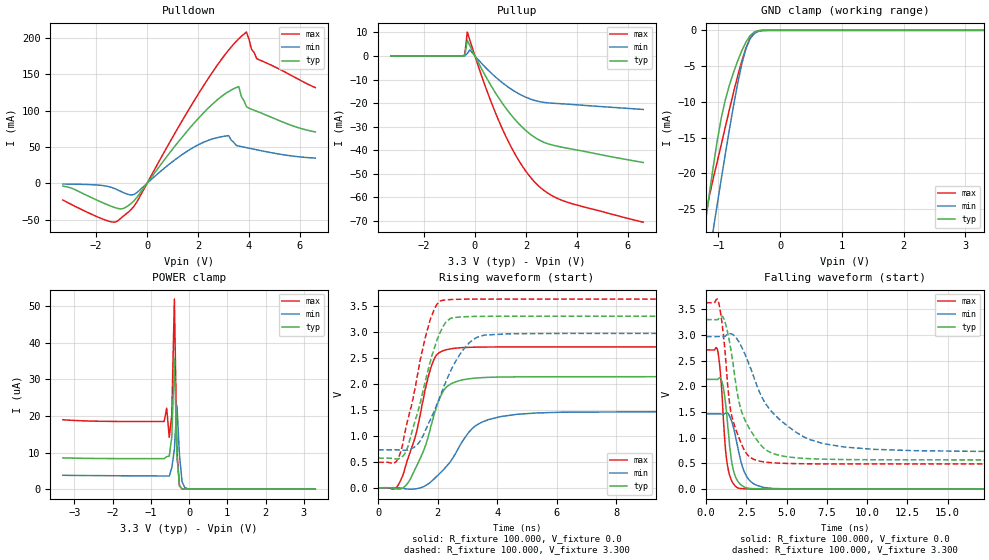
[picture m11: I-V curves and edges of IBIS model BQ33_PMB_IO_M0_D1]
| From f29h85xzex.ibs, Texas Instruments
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|   Model BQ33_PMB_IO_M0_D1
[Model]   BQ33_PMB_IO_M0_D1
Model_type   I/O
Polarity   Non-Inverting
Enable   Active-Low
Vinl =   0.990V
Vinh =   2.310V
Vmeas =  1.650V
Cref =   100.000pF
Vref =   0.0V
|   typ   min   max
C_comp   1.646pF   1.624pF   1.799pF
[Model Spec]
Vinh   2.310V   2.079V   2.541V
Vinl   0.990V   0.891V   1.089V
[Temperature Range]   30   155   -40
[Voltage Range]   3.300V   2.970V   3.630V
[Pullup Reference]   3.300V   2.970V   3.630V
[Pulldown Reference]   0.0V   0.0V   0.0V
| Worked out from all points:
|   slope of the pulldown table from 0 to 0.495 V, typ, clamps not added: 20.8 ohm
|   slope of the pullup table from 0 to 0.495 V, typ, clamps not added: 49.3 ohm
|   GND clamp passes 1 mA (typ) near -0.51 V on its own axis
|   rising waveform, R_fixture 100.000, V_fixture 0.0: 20-80 % time 760ps typ, 1.13ns min, 713ps max; typ from 0 V to 2.14 V
|   rising waveform, R_fixture 100.000, V_fixture 3.300: 20-80 % time 773ps typ, 1.05ns min, 715ps max; typ from 0.57 V to 3.3 V
|   falling waveform, R_fixture 100.000, V_fixture 0.0: 20-80 % time 459ps typ, 715ps min, 378ps max; typ from 2.14 V to 0 V
|   falling waveform, R_fixture 100.000, V_fixture 3.300: 20-80 % time 1.3ns typ, 2.73ns min, 820ps max; typ from 3.3 V to 0.57 V
[Pulldown]
|Voltage   I(typ)   I(min)   I(max)
-3.3V     -3.922mA   -895.2uA   -22.93mA
-1.4V     -31.61mA   -5.503mA   -53.04mA
-700mV    -29.75mA   -15.57mA   -38.53mA
-400mV    -19.4mA    -12.77mA   -25.68mA
1.6V      72.96mA    44.8mA     99.38mA
2.8V      116.3mA    63.33mA    164.9mA
3.2V      126.4mA    65.74mA    183.5mA
3.6V      133.3mA    51.35mA    199.2mA
3.9V      105.6mA    49.16mA    208.3mA
4.1V      102mA      47.7mA     184.6mA
4.3V      99.3mA     46.24mA    171.8mA
6.6V      70.82mA    34.77mA    131.8mA
[Pullup]
|Voltage   I(typ)   I(min)   I(max)
-3.3V     -1.722nA   12.42nA    1.362nA
-500mV    17.15nA    18.01nA    59.06nA
-400mV    178uA      374.8nA    408.1uA
-300mV    6.695mA    1.073mA    10.14mA
-200mV    4.421mA    2.585mA    6.742mA
400mV     -8.225mA   -4.706mA   -12.71mA
1V        -18.86mA   -10.69mA   -29.11mA
1.7V      -28.5mA    -15.89mA   -44mA
2.3V      -34.18mA   -18.71mA   -52.97mA
2.8V      -37.02mA   -19.82mA   -57.77mA
3.5V      -38.88mA   -20.34mA   -61.58mA
6.6V      -45.18mA   -22.68mA   -70.51mA
[GND_clamp]
|Voltage   I(typ)   I(min)   I(max)
-3.3V     -172.4mA   -157.9mA   -199.3mA
-1.223V   -27.66mA   -35.7mA    -26.88mA
-1.156V   -23.42mA   -31.92mA   -23.54mA
-1.089V   -19.35mA   -28.18mA   -20.9mA
-1.022V   -15.58mA   -24.48mA   -18.47mA
-955mV    -12.3mA    -20.84mA   -16.02mA
-821mV    -7.634mA   -13.8mA    -11.02mA
-620mV    -2.823mA   -4.656mA   -4.248mA
-553mV    -1.627mA   -2.518mA   -2.447mA
-419mV    -233.8uA   -454.3uA   -289uA
-218mV    -985nA     -9.253uA   -449.5nA
3.3V      0A         0A         0A
[POWER_clamp]
|Voltage   I(typ)   I(min)   I(max)
-3.3V     8.55uA     3.797uA    18.96uA
-653mV    8.339uA    3.596uA    18.47uA
-586mV    8.872uA    3.591uA    22.11uA
-519mV    9.031uA    3.588uA    14.17uA
-452mV    14.26uA    5.833uA    20.33uA
-385mV    35.62uA    10.82uA    51.91uA
-318mV    9.151uA    22.94uA    10.03uA
-251mV    942nA      9.217uA    856.3nA
-184mV    84.85nA    2.059uA    62.73nA
-117mV    8.015nA    524.6nA    4.599nA
-50mV     1.476nA    168.6nA    663.4pA
3.3V      0A         0A         0A
[Ramp]
| variable   typ   min   max
dV/dt_r   1.282/0.762n   0.879/1.130n   1.626/0.713n
dV/dt_f   1.638/1.297n   1.344/2.724n   1.884/0.822n
R_load = 100.000
[Rising Waveform]
R_fixture= 100.000
V_fixture= 0.0
V_fixture_min= 0.0
V_fixture_max= 0.0
|time   V(typ)   V(min)   V(max)
0s        81.49uV    68.2uV     93.5uV
760ps     -20.09mV   -4.77mV    146.4mV
1.44ns    591.1mV    3.166mV    1.47V
1.67ns    948.6mV    70.16mV    2.111V
1.93ns    1.491V     199.1mV    2.528V
2.29ns    1.935V     408mV      2.655V
2.87ns    2.08V      926.3mV    2.697V
3.72ns    2.125V     1.314V     2.708V
6.13ns    2.136V     1.453V     2.71V
100ns     2.137V     1.465V     2.71V
[Rising Waveform]
R_fixture= 100.000
V_fixture= 3.300
V_fixture_min= 2.970
V_fixture_max= 3.630
|time   V(typ)   V(min)   V(max)
0s        569.7mV    730.6mV    489.7mV
580ps     556.5mV    731.1mV    490.7mV
900ps     661.6mV    721.4mV    1.06V
1.35ns    1.49V      851.4mV    2.255V
1.77ns    2.467V     1.329V     3.268V
2.15ns    3.072V     1.861V     3.603V
2.48ns    3.265V     2.3V       3.622V
3.33ns    3.297V     2.897V     3.629V
4.45ns    3.3V       2.963V     3.63V
100ns     3.3V       2.97V      3.63V
[Falling Waveform]
R_fixture= 100.000
V_fixture= 0.0
V_fixture_min= 0.0
V_fixture_max= 0.0
|time   V(typ)   V(min)   V(max)
0s        2.137V     1.465V     2.71V
700ps     2.136V     1.465V     2.722V
990ps     2.084V     1.464V     1.829V
1.17ns    1.767V     1.47V      895.5mV
1.36ns    1.175V     1.472V     403.7mV
1.66ns    411.5mV    1.243V     122.2mV
2.17ns    82.46mV    530.9mV    12.69mV
2.95ns    10.18mV    105.7mV    3.702mV
4.97ns    1.777mV    6.826mV    846uV
100ns     275.3nV    4.001uV    153.9nV
[Falling Waveform]
R_fixture= 100.000
V_fixture= 3.300
V_fixture_min= 2.970
V_fixture_max= 3.630
|time   V(typ)   V(min)   V(max)
0s        3.3V       2.97V      3.63V
750ps     3.305V     2.97V      3.669V
1.09ns    3.326V     2.968V     2.946V
1.5ns     2.779V     3.027V     1.569V
2.05ns    1.69V      2.861V     988.1mV
2.69ns    1.179V     2.407V     631.3mV
3.82ns    743.4mV    1.608V     522mV
6.42ns    593.4mV    967.6mV    493.5mV
12.92ns   570.6mV    749.5mV    489.9mV
100ns     569.6mV    730.5mV    489.6mV
